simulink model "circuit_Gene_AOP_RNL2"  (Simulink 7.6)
settings: Solver=ode15s  StartTime=0.0  StopTime=3  RelTol=1e-3
InitFcn:
  | clc
StopFcn:
  | % lecture du fichier binaire
  | load gen_sin.mat
  | 
  | % trace de la tension et du courant d’induit
  | plot(x(1,:),x(2,:),x(1,:),x(3,:))
  | title('Entrée/sortie - ampli op résistance non linéaire')
  | grid
libraries: fl_lib x4, MaLibrairieElectrical_lib x3, nesl_utility x3

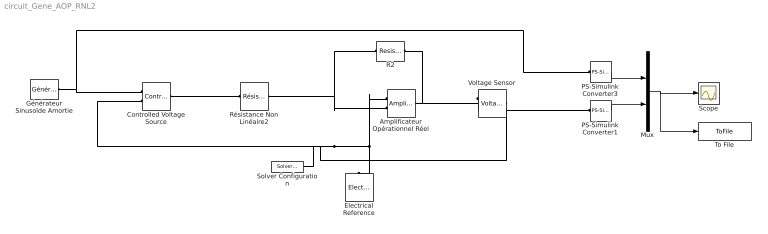
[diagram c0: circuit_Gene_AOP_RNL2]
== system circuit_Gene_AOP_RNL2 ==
  Amplificateur Opérationnel Réel : MaLibrairieElectrical_lib/Amplificateur Opérationnel Réel  DialogController=NetworkEngine.DynNeDlgSource  SystemSampleTime=-1  A=1e+6  Re=1e+6 Ohm  Rs=100 Ohm  Vsat=15 V  ie_Log=off  eps_Log=off  is_Log=off  vs_Log=off  LocalVarNames=|ie|eps|is|vs  LocalVarDescs=|ie|eps|is|vs  LocalVarLogging=[0 0 0 0]
  Controlled Voltage Source : fl_lib/Electrical/Electrical Sources/Controlled Voltage Source  DialogController=NetworkEngine.DynNeDlgSource  SystemSampleTime=-1  i_Log=off  v_Log=off  LocalVarNames=|i|v  LocalVarDescs=|i|v  LocalVarLogging=[0 0]
  Electrical Reference : fl_lib/Electrical/Electrical Elements/Electrical Reference  DialogController=NetworkEngine.DynNeDlgSource  SystemSampleTime=-1  i_Log=off  LocalVarNames=|i  LocalVarDescs=|i  LocalVarLogging=0
  Générateur Sinusoïde Amortie : MaLibrairieElectrical_lib/Générateur Sinusoïde Amortie  DialogController=NetworkEngine.DynNeDlgSource  SystemSampleTime=-1  biais=0  w=6.2832 1/s  Amp=5  phi=0 rad  a=2  LocalVarLogging=[]
  Mux : Mux  Inputs=2
  PS-Simulink Converter1 : nesl_utility/PS-Simulink Converter  DialogController=NetworkEngine.DynNeUtilDlgSource  SystemSampleTime=-1  PhysicalDomain=network_engine_domain  LeftPortType=input  RightPortType=output  SubClassName=ps_output  Unit=1  AffineConversion=off
  PS-Simulink Converter3 : nesl_utility/PS-Simulink Converter  DialogController=NetworkEngine.DynNeUtilDlgSource  SystemSampleTime=-1  PhysicalDomain=network_engine_domain  LeftPortType=input  RightPortType=output  SubClassName=ps_output  Unit=1  AffineConversion=off
  R2 : fl_lib/Electrical/Electrical Elements/Resistor  DialogController=NetworkEngine.DynNeDlgSource  SystemSampleTime=-1  R=10 kOhm  i_Log=off  v_Log=off  LocalVarNames=|i|v  LocalVarDescs=|i|v  LocalVarLogging=[0 0]
  Résistance Non Linéaire2 : MaLibrairieElectrical_lib/Résistance Non Linéaire2  DialogController=NetworkEngine.DynNeDlgSource  SystemSampleTime=-1  R0=20 kOhm  K=200 V/A^2  i_Log=off  v_Log=off  LocalVarNames=|i|v  LocalVarDescs=|i|v  LocalVarLogging=[0 0]
  Scope : Scope
  Solver Configuration : nesl_utility/Solver Configuration  DialogController=NetworkEngine.DynNeUtilDlgSource  SystemSampleTime=-1  PhysicalDomain=network_engine_domain  LeftPortType=input  RightPortType=generic  SubClassName=solver  Accelerate=off  Profile=off  ResidualTolerance=1e-9  MaxNonlinIter=3  MaxModeIter=2  DoFixedCost=off  UseLocalSampling=off  DoDC=off  LinearAlgebra=Sparse  LocalSolverSampleTime=.001  LocalSolverChoice=NE_BACKWARD_EULER_ADVANCER  UseLocalSolver=off
  To File : ToFile  Filename=gen_sin  MatrixName=x
  Voltage Sensor : fl_lib/Electrical/Electrical Sensors/Voltage Sensor  DialogController=NetworkEngine.DynNeDlgSource  SystemSampleTime=-1  i1_Log=off  v1_Log=off  LocalVarNames=|i1|v1  LocalVarDescs=|i1|v1  LocalVarLogging=[0 0]
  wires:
  Mux/1 -> Scope/1, To File/1
  PS-Simulink Converter1/1 -> Mux/2
  PS-Simulink Converter3/1 -> Mux/1
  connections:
  R2/RConn1 -- Amplificateur Opérationnel Réel/RConn1 -- Voltage Sensor/LConn1
  Générateur Sinusoïde Amortie/RConn1 -- Controlled Voltage Source/RConn1 -- PS-Simulink Converter3/LConn1
  Voltage Sensor/RConn1 -- PS-Simulink Converter1/LConn1
  Controlled Voltage Source/RConn2 -- Voltage Sensor/RConn2 -- Electrical Reference/LConn1 -- Amplificateur Opérationnel Réel/LConn1 -- Solver Configuration/RConn1
  Résistance Non Linéaire2/RConn1 -- R2/LConn1 -- Amplificateur Opérationnel Réel/LConn2
  Controlled Voltage Source/LConn1 -- Résistance Non Linéaire2/LConn1
